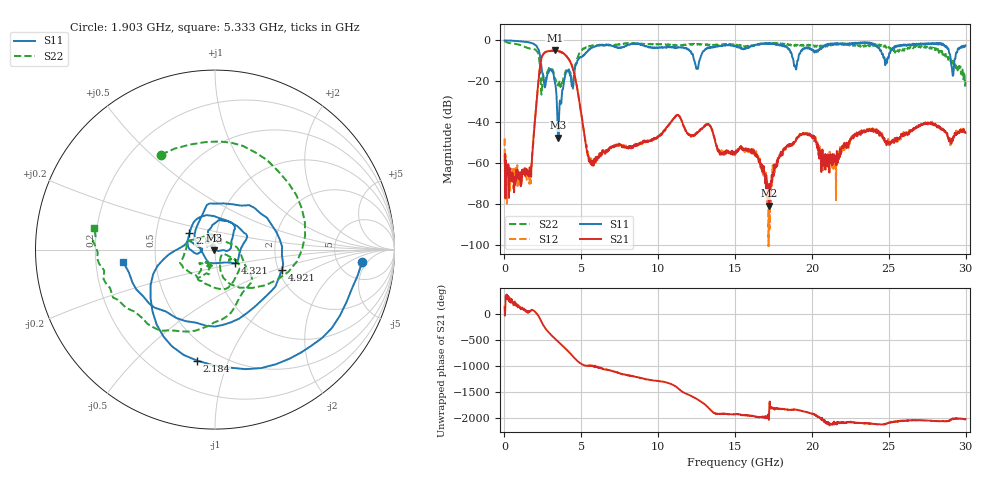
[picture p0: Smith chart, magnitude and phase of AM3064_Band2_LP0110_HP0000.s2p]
# Hz S DB R 50.0
!freq dBS11 angS11 dBS21 angS21 dBS12 angS12 dBS22 angS22
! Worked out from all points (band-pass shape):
!   1600 points, 10 MHz to 29.98 GHz, reference 50 ohm
!   highest |S21| = -4.94 dB at 3.271 GHz (marker M1); lowest = -80.8 dB at 17.2 GHz (marker M2)
!   |S21| within 3 dB of the highest: 2.443 GHz to 4.061 GHz (1.618 GHz wide, 49.8 % of centre)
!   lowest |S11| = -47.5 dB at 3.515 GHz (marker M3), VSWR 1.01, Z = 49.6 - j0.181 ohm
!   |S11| at or under -10 dB: 2.361 GHz to 4.743 GHz (2.382 GHz wide, 67.1 % of centre); 12.36 GHz to 12.67 GHz (317 MHz wide, 2.53 % of centre); 18.8 GHz to 19.05 GHz (253.4 MHz wide, 1.34 % of centre)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
!   |S22| runs from -26.5 to -0.2 dB; largest |S21 - S12| = 0.023
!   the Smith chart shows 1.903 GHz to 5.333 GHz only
!   S11 on the Smith chart (normalised r, x): 1.903 GHz: 8.59, -3.76; 2.184 GHz: 0.38, -0.78; 2.878 GHz: 0.74, +0.14; 4.321 GHz: 1.24, -0.19; 4.921 GHz: 2.09, -0.56; 5.333 GHz: 0.32, -0.06
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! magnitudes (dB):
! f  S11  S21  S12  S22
! 10 MHz  0.0  -56.4  -48.0  -0.2
! 1.566 GHz  -0.9  -64.7  -64.7  -3.8
! 1.903 GHz  -1.7  -46.6  -47.1  -4.3
! 2.184 GHz  -4.1  -22.0  -22.0  -6.3
! 2.878 GHz  -15.5  -5.2  -5.3  -13.8
! 3.271 GHz  -20.3  -4.9  -5.0  -19.0
! 3.515 GHz  -47.5  -5.3  -5.3  -21.8
! 4.321 GHz  -17.4  -11.1  -11.1  -17.1
! 4.921 GHz  -8.2  -32.1  -32.0  -5.6
! 5.015 GHz  -8.2  -36.7  -36.8  -5.1
! 5.333 GHz  -5.7  -52.7  -51.0  -3.3
! 10 GHz  -3.6  -47.1  -46.9  -1.9
! 11.27 GHz  -3.4  -36.3  -36.3  -2.6
! 15 GHz  -2.7  -54.4  -55.6  -2.1
! 16.28 GHz  -2.3  -54.6  -56.0  -2.4
! 17.2 GHz  -1.6  -80.8  -77.2  -1.7
! 18.3 GHz  -2.7  -52.3  -51.9  -2.1
! 19.99 GHz  -4.4  -46.9  -47.1  -2.3
! 21.43 GHz  -2.1  -58.6  -58.5  -1.7
! 23.31 GHz  -1.0  -44.2  -44.9  -2.6
! 25 GHz  -8.1  -49.9  -51.2  -3.2
! 29.98 GHz  -2.5  -45.2  -45.4  -20.2
